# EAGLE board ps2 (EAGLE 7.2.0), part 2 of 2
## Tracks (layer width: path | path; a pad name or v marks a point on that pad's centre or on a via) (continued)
KNOCKER+ (continued)
  Top 0.254: R18.1 99.21,12.23 100.36,12.23 103.33,15.2 114.19,15.2 115.67,13.72 R45.2
  Bottom 0.254: OK7.1 121.16,22.06 117.16,18.06 117.16,15.09 115.79,13.72 R45.2
KNOCKER-  (via drill 0.61)
  Top 0.254: 124.3,14.92 123.1,13.72 R48.1 | 124.3,14.92 127.33,17.95 127.33,24.12 126.64,24.8 125.84,24.8 125.62,24.57 120.81,24.57 119.79,25.6 118.64,25.6 OK7.2 | v8.12,27.77 6.63,29.26 6.63,34.4 2.63,38.41 2.63,38.86 T3.C | v31.77,15.66 33.15,15.09 50.41,15.09 54.41,11.09 66.75,11.09 67.32,11.66 67.32,14.4 65.95,15.77 64.35,15.77 63.78,16.46 63.78,18.75 64.81,19.77 69.84,19.77 73.15,16.46 73.15,12 76.35,8.8 76.35,5.83 v77.84,4.34 | v96.24,4.34 99.44,4.34 99.61,4.17 | 99.61,4.17 101.73,2.06 R10.2 | v99.67,4.23 99.61,4.17 | 124.3,14.92 127.67,11.54 v127.67,11.43 | v121.84,8.91 121.84,11.09 120.93,12 113.96,12 112.47,10.52 C9.2
  Bottom 0.254: v8.12,27.77 11.2,24.69 22.75,24.69 v31.77,15.66 | v96.24,4.34 v77.84,4.34 | v99.67,4.23 102.3,6.86 112.81,6.86 113.39,7.43 113.39,8.34 112.47,9.26 112.47,10.4 C9.2 | v127.67,11.43 127.1,11.43 124.24,8.57 122.19,8.57 v121.84,8.91
KNOCKER_TRIGGER  (via drill 0.61)
  Top 0.254: v18.63,68.01 18.63,77.15 20.8,79.32 21.83,79.32 22.75,78.41 22.75,77.72 23.66,76.81 24.35,76.81 v26.86,74.3 | v30.29,64.58 31.77,63.09 31.77,59.44 33.26,57.95 FRDM1.D6
  Bottom 0.254: v18.63,68.01 15.66,65.04 15.66,54.86 12.46,51.66 12.46,47.43 R37.1 | v26.86,74.3 26.86,70.98 30.29,67.55 v30.29,64.58
MOSFETIN2
  Top 0.254: IC2.4 100.36,23.66 111.56,23.66 113.5,25.6 OK7.4
MOSFETIN3
  Top 0.254: OK7.6 108.36,25.6 107.33,25.6 106.3,24.57 101.84,24.57 100.36,26.06 IC2.5
MOSFETIN4
  Top 0.254: IC2.6 100.36,28.69 103.33,25.72 OK7.8
MOSFETIN5
  Top 0.254: IC2.7 100.36,31.32 105.16,31.32 107.21,33.38 114.41,33.38 118.53,37.49 OK8.2
MOSFETIN6
  Top 0.254: OK8.4 109.84,33.83 100.36,33.83 IC2.8
MOSFETIN7
  Top 0.254: IC2.9 100.36,36.35 107.21,36.35 108.36,37.49 OK8.6
MOSFETIN8
  Top 0.254: IC2.10 102.07,38.86 103.33,37.6 OK8.8
MOSFETIN9
  Top 0.254: IC2.11 100.36,41.49 101.61,41.49 103.67,43.55 107.44,43.55 112.24,48.35 117.5,48.35 118.53,49.38 OK9.2
MOSFETIN10
  Top 0.254: IC2.12 100.36,44.01 107.21,44.01 112.58,49.38 113.5,49.38 OK9.4
MOSFETIN11
  Top 0.254: IC2.13 100.36,46.52 105.5,46.52 108.36,49.38 OK9.6
MOSFETIN12
  Top 0.254: IC2.14 100.36,49.03 102.98,49.03 103.33,49.38 OK9.8
MOSFETIN13  (via drill 0.61)
  Top 0.254: v101.04,52.46 100.24,51.66 95.56,51.66 IC2.15
  Bottom 0.254: v101.04,52.46 102.3,53.72 102.3,58.86 104.93,61.49 104.93,66.06 105.5,66.64 116.59,66.64 117.61,65.61 117.61,62.41 118.53,61.49 OK10.2
MOSFETIN14  (via drill 0.61)
  Top 0.254: v106.07,59.66 101.73,55.32 99.67,55.32 96.47,52.12 94.18,52.12 92.81,53.49 92.81,53.84 IC3.28
  Bottom 0.254: v106.07,59.66 111.78,59.66 113.5,61.38 OK10.4
MOSFETIN15
  Top 0.254: IC3.1 100.36,53.95 101.61,53.95 108.36,60.69 108.36,61.38 OK10.6
MOSFETIN16
  Top 0.254: IC3.2 100.36,56.46 100.36,56.81 103.33,59.78 103.33,61.38 OK10.8
MOSFETIN17
  Bottom 0.254: IC3.3 100.36,58.98 100.36,59.32 102.3,61.27 102.3,66.06 104.93,68.69 113.96,68.69 118.53,73.27 OK11.2
MOSFETIN18  (via drill 0.61)
  Top 0.254: v102.64,68.01 102.64,68.58 104.93,70.87 104.93,77.95 105.96,78.98 110.98,78.98 112.47,77.5 112.47,74.3 113.5,73.27 OK11.4
  Bottom 0.254: v102.64,68.01 99.67,68.01 98.64,66.98 98.64,63.55 100.24,61.95 100.24,61.49 IC3.4
MOSFETIN19
  Top 0.254: IC3.5 100.36,64.01 100.36,64.47 107.67,71.78 107.67,72.58 108.36,73.27 OK11.6
MOSFETIN20
  Top 0.254: IC3.6 100.36,66.64 100.36,66.98 103.33,69.95 103.33,73.27 OK11.8
MOSFETIN21
  Bottom 0.254: IC3.7 100.36,69.15 108.36,69.15 112.47,73.27 112.47,78.3 118.53,84.35 118.53,85.04 OK12.2
MOSFETIN22
  Bottom 0.254: IC3.8 100.36,71.67 103.21,71.67 104.47,72.92 104.47,79.9 107.56,82.98 111.44,82.98 113.5,85.04 OK12.4
MOSFETIN23
  Top 0.254: IC3.9 100.36,74.18 100.36,74.64 102.3,76.58 102.3,78.41 108.36,84.47 108.36,85.04 OK12.6
MOSFETIN24
  Top 0.254: IC3.10 100.36,76.81 100.36,77.15 105.73,82.53 105.73,83.67 104.24,83.67 OK12.8
MOSFETOUT1  (via drill 0.61)
  Top 1.575: Q7A.2 145.03,6.86 150.53,12.8 v150.53,15.54
  Bottom 1.575: v150.53,15.54 153.28,18.75 JP10.1
MOSFETOUT2
  Bottom 1.575: Q7B.2 130.81,5.71 130.81,9.53 136.53,9.53 137.16,10.16 137.16,13.34 136.53,13.97 136.53,16.51 148.59,16.51 150.42,18.52 JP10.2
MOSFETOUT3
  Bottom 1.575: Q7C.2 144.15,9.53 147.71,9.53 149.39,11.54 152.82,15.2 153.62,16.12 155.87,18.82 155.87,20.79 154.42,22.05 JP10.3
MOSFETOUT4
  Bottom 1.575: Q7D.2 130.81,13.97 130.81,18.41 147.32,18.41 150.72,22.16 151.36,22.16 JP10.4
MOSFETOUT5
  Top 1.575: Q8A.2 141.6,20.95 141.6,19.68 143.51,17.78 154.94,17.78 156.21,19.05 156.21,22.86 154.31,24.77 JP10.5
MOSFETOUT6
  Bottom 1.575: Q8B.2 128.91,22.86 128.91,25.4 150.5,25.4 151.13,24.77 JP10.6
MOSFETOUT7  (via drill 0.61)
  Top 1.575: v156.21,35.56 156.21,29.21 154.31,27.3 JP10.7 | v144.15,36.83 140.97,33.66 140.97,30.48 Q8C.2
  Bottom 1.575: v156.21,35.56 154.94,36.83 v144.15,36.83
MOSFETOUT8
  Bottom 1.575: Q8D.2 128.91,31.75 128.91,27.3 151.13,27.3 JP10.8
MOSFETOUT9
  Bottom 1.575: Q9A.2 141.48,34.92 154.31,34.92 156.21,33.02 156.21,29.84 154.31,29.84 JP10.9
MOSFETOUT10  (via drill 0.61)
  Top 1.575: v142.88,33.02 144.78,34.92 147.32,34.92 148.34,33.66 148.34,31.75 149.99,29.84 151.13,29.84 JP10.10
  Bottom 1.575: v142.88,33.02 139.06,33.02 134.62,37.47 132.72,37.47 128.78,40.77 Q9B.2
MOSFETOUT11
  Top 1.575: JP10.11 153.9,32.61 153.96,33.83 151.02,37.21 150.77,37.71 150.75,47.12 149.61,49.02 146.94,49.02 146.05,47.37 143.89,46.35 141.48,47.75 Q9C.2
MOSFETOUT12  (via drill 0.61)
  Top 1.575: v148.48,41.47 148.48,36.8 151.33,33.38 151.36,32.5 JP10.12
  Bottom 1.575: v148.48,41.47 148.46,43.56 147.83,44.83 146.3,44.83 144.91,46.61 132.21,46.61 128.78,49.91 Q9D.2
MOSFETOUT13
  Top 1.575: Q10A.2 156.21,46.99 155.57,46.99 152.4,50.16 152.4,57.15 154.31,59.05 JP11.1
MOSFETOUT14
  Top 1.575: Q10B.2 141.6,57.78 141.6,57.15 143.51,55.24 147.32,55.24 151.13,59.05 JP11.2
MOSFETOUT15  (via drill 0.61)
  Top 1.575: v154.31,55.24 156.21,57.15 156.21,60.33 154.31,62.23 JP11.3
  Bottom 1.575: v154.31,55.24 128.91,55.24 128.91,59.69 Q10C.2
MOSFETOUT16
  Bottom 1.575: JP11.4 151.13,62.23 147.32,62.23 146.69,62.87 133.99,62.87 128.91,67.94 128.91,69.22 Q10D.2
MOSFETOUT17  (via drill 0.61)
  Top 1.575: v147.96,59.69 147.96,61.59 144.78,64.77 v138.89,64.77
  Bottom 1.575: v147.96,59.69 150.5,57.15 156.21,57.15 156.21,62.23 154.31,64.14 JP11.5 | Q11A.2 128.84,76.33 132.72,73.03 133.35,72.45 133.35,69.85 133.39,69.85 133.39,69.72 135.56,67.44 135.56,65.95 136.82,64.81 v138.89,64.77
MOSFETOUT18
  Bottom 1.575: JP11.6 151.13,64.77 143.51,64.77 141.48,66.29 Q11B.2
MOSFETOUT19  (via drill 0.61)
  Top 1.575: v149.22,75.56 147.32,75.56 144.78,73.03 143.51,73.03 141.48,75.18 Q11C.2
  Bottom 1.575: v149.22,75.56 149.86,74.93 156.21,74.93 156.21,68.58 154.94,67.31 154.31,67.31 JP11.7
MOSFETOUT20
  Bottom 1.575: Q11D.2 128.79,84.99 128.79,83.96 132.08,80.64 133.99,78.74 133.99,76.83 134.62,76.83 139.7,71.75 147.32,71.75 149.22,69.85 149.22,67.31 151.13,67.31 JP11.8
MOSFETOUT21  (via drill 0.61)
  Top 1.575: Q12A.2 144.78,92.08 v149.22,87.63 | v154.94,76.83 156.21,75.56 156.21,71.12 154.31,69.22 JP11.9
  Bottom 1.575: v149.22,87.63 149.22,80.64 150.5,79.38 150.5,76.83 v154.94,76.83
MOSFETOUT22  (via drill 0.61)
  Top 1.575: v146.69,92.71 151.13,88.27 151.13,74.3 149.22,72.39 149.22,71.12 151.13,69.22 JP11.10
  Bottom 1.575: Q12B.2 131.44,92.71 v146.69,92.71
MOSFETOUT23  (via drill 0.61)
  Top 1.575: v153.03,78.74 153.03,76.2 153.67,75.56 153.67,72.39 JP11.11
  Bottom 1.575: v153.03,78.74 152.4,79.38 152.4,85.09 Q12C.2
MOSFETOUT24
  Bottom 1.575: Q12D.2 141.6,85.09 141.6,80.64 146.69,80.64 147.96,79.38 147.96,76.83 147.32,76.2 147.32,73.66 148.59,73.66 149.86,72.39 151.13,72.39 JP11.12
N$1  (via drill 0.61)
  Top 0.254: v96.24,24.57 96.24,33.03 93.95,35.32 89.72,35.32 89.15,35.89 89.15,36.69 88.47,37.38 86.75,37.38 80.24,43.89 79.78,43.89 IC1.17
  Bottom 0.254: v96.24,24.57 92.81,21.14 IC2.26
N$2
  Top 0.254: IC2.17 92.7,44.01 91.21,44.01 89.15,46.06 89.15,50.98 90.53,52.35 90.53,56.69 92.7,58.86 IC3.26
N$3  (via drill 0.61)
  Top 0.254: v83.67,56.01 83.67,67.44 83.78,67.55 83.78,74.3 v83.33,74.75 | v95.33,79.32 95.33,80.58 94.18,81.72 92.81,81.72 IC3.17
  Bottom 0.254: v83.67,56.01 80.81,58.86 79.78,58.86 IC4.26 | v83.33,74.75 86.3,77.72 93.73,77.72 v95.33,79.32
N$4
  Bottom 0.254: R18.2 99.21,2.06 99.21,2.52 103.1,6.4 114.07,6.4 117.96,10.29 IC11.3
N$5
  Top 0.254: OK15.1 16.92,70.29 15.89,70.29 14.86,69.27 14.06,69.27 12,71.32 12,71.55 R39.1
N$6  (via drill 0.61)
  Top 0.254: v103.44,4.23 102.41,5.26 95.9,5.26 95.33,4.69 95.33,4 96.58,2.74 96.58,2.06 R6.1 | IC11.4 115.44,10.29 113.73,10.29 112.36,8.91 112.01,8.91 106.98,3.89 C5.+
  Bottom 0.254: v103.44,4.23 106.64,4.23 C5.+
N$8  (via drill 0.61)
  Top 0.254: v2.86,70.75 2.86,68.69 1.26,67.09 1.26,32.92 4.34,29.83 4.34,25.95 2.06,23.66 R38.1 | v2.86,83.33 2.86,85.84 1.83,86.87 R47.2 1.83,86.98 1.83,87.55 10.74,96.47 10.74,96.93 T5.C
  Bottom 0.254: v2.86,83.33 v2.86,70.75
N$9
  Bottom 0.254: R37.2 2.63,45.83 5.03,43.55 5.03,38.86 T3.B
N$10
  Top 0.254: OK13.1 10.97,26.4 10.97,24.8 12.12,23.66 R38.2
N$11
  Top 0.254: R49.2 12,69.04 12,65.15 14.4,62.75 OK15.3
N$12
  Bottom 0.254: T6.B 5.03,33.72 4.57,33.72 2.97,32.12 2.06,32.12 1.26,32.92 1.26,68.58 1.71,69.04 R49.1
N$13
  Top 0.254: R44.2 1.83,79.32 1.83,79.78 8.8,86.75 8.8,92.47 10.74,94.41 T5.B
N$14
  Top 0.254: R44.1 12,79.32 12,81.72 R41.1 12,81.84 12,82.87 17.49,88.35 17.49,94.53 15.43,96.58 15.43,96.93 T4.C
N$15  (via drill 0.61)
  Top 0.254: v30.52,20.34 31.77,20.34 32.58,19.55 32.58,16.92 33.72,15.54 50.63,15.54 54.18,12 v66.41,12 | v83.21,12.34 91.78,12.34 D1.A
  Bottom 0.254: v30.52,20.34 22.29,28.57 16.92,28.57 10.06,35.43 4.57,35.43 2.97,33.83 2.63,33.83 T6.C | v66.41,12 71.32,12 73.5,9.83 K1.16 73.61,9.83 74.87,11.09 81.95,11.09 v83.21,12.34
N$16
  Top 0.254: K1.4 81.15,2.29 76.81,6.63 76.81,13.03 JP9.2
N$17
  Top 0.254: R2.1 77.04,36.35 79.67,36.35 IC1.20
N$18
  Top 0.254: R3.1 90.18,36.35 92.7,36.35 IC2.20
N$19
  Top 0.254: R4.1 89.95,74.18 92.7,74.18 IC3.20
N$20
  Top 0.254: R5.1 77.27,74.18 79.67,74.18 IC4.20
N$21
  Bottom 0.254: FRDM1.A0 35.78,9.6 35.78,6.06 35.55,5.83 35.55,2.4 36.35,1.6 56.81,1.6 59.44,4.23 66.06,4.23 67.21,5.37 JP7.1
N$22  (via drill 0.61)
  Top 0.254: v55.78,21.14 49.15,21.14 44.46,25.83 44.01,25.83 IC5.3
  Bottom 0.254: v55.78,21.14 58.64,18.29 58.64,16.57 59.78,15.43 64.69,15.43 67.21,17.95 67.21,18.29 OK1.15
N$23
  Bottom 0.254: OK1.13 61.15,18.29 55.44,24 38.18,24 36.35,25.83 IC5.6
N$24
  Top 0.254: IC5.11 36.69,18.29 38.41,16.57 41.83,16.57 42.86,17.6 42.86,19.32 44.01,20.46 51.32,20.46 53.61,18.17 53.61,16.46 54.18,15.89 54.98,15.89 57.15,18.06 OK1.11
N$25
  Top 0.254: IC5.14 44.35,18.29 46.06,20 50.29,20 52.01,18.29 OK1.9
N$26
  Top 0.254: FRDM1.PTE20 35.89,12.23 36.46,12.23 38.86,14.63 50.06,14.63 56.81,7.89 64.01,7.89 65.95,5.94 65.95,2.17 65.27,1.6 64.12,1.6 63.44,2.29 63.44,3.43 62.64,4.23 61.27,4.23 JP7.8
N$27  (via drill 0.61)
  Top 0.254: v57.49,34.75 47.43,34.75 44.35,37.83 44.01,37.83 IC6.3 | v66.06,32.69 66.06,32.12 67.21,30.98 67.21,30.29 OK2.15
  Bottom 0.254: v57.49,34.75 58.06,34.75 60.12,32.69 v66.06,32.69
N$28  (via drill 0.61)
  Top 0.254: v56.58,33.83 v48.12,33.83
  Bottom 0.254: v48.12,33.83 40.8,33.83 36.8,37.83 36.35,37.83 IC6.6 | v56.58,33.83 58.29,33.83 61.84,30.29 62.18,30.29 OK2.13
N$29  (via drill 0.61)
  Top 0.254: v45.26,32.35 55.09,32.35 57.15,30.29 OK2.11
  Bottom 0.254: v45.26,32.35 38.86,32.35 36.8,30.29 36.35,30.29 IC6.11
N$30
  Top 0.254: OK2.9 50.41,31.89 46.06,31.89 44.46,30.29 44.01,30.29 IC6.14
N$31  (via drill 0.61)
  Top 0.254: v48.35,44.12 48.35,45.38 IC7.3
  Bottom 0.254: v48.35,44.12 54.06,44.12 55.66,42.52 55.66,37.83 59.44,34.06 65.38,34.06 65.95,34.63 65.95,39.32 67.21,40.58 67.21,42.06 OK3.15
N$32
  Bottom 0.254: OK3.13 62.18,42.18 61.15,42.18 57.38,45.95 40.12,45.95 36.35,49.72 IC7.6
N$33  (via drill 0.61)
  Top 0.254: v37.26,45.95 36.35,45.03 36.35,42.18 IC7.11
  Bottom 0.254: v37.26,45.95 39.43,45.95 39.89,45.49 56.69,45.49 57.26,44.92 57.26,42.29 57.15,42.18 OK3.11
N$34
  Top 0.254: FRDM1.PTE21 38.41,12.23 38.98,12.23 40.92,14.17 49.84,14.17 56.58,7.43 62.75,7.43 64.69,5.49 JP7.3
N$35
  Bottom 0.254: IC7.14 44.01,42.06 44.46,42.06 46.06,40.46 50.41,40.46 52.01,42.06 OK3.9
N$36
  Top 0.254: IC8.3 42.98,70.18 43.43,70.18 45.03,71.78 50.06,71.78 57.84,64.01 68.01,64.01 69.49,62.52 OK4.15
N$37
  Bottom 0.254: OK4.13 64.35,62.52 63.32,62.52 57.72,68.12 53.49,68.12 52.46,67.09 38.29,67.09 35.32,70.07 IC8.6
N$38
  Top 0.254: JP6.2 50.86,4 50.86,5.6 49.95,6.51 49.72,6.51 47.43,8.8 47.43,10.17 46.06,11.54 46.06,12.12 FRDM1.PTE29
N$39  (via drill 0.61)
  Top 0.254: v48.58,59.89 37.6,59.89 35.32,62.18 35.32,62.41 IC8.11
  Bottom 0.254: v48.58,59.89 57.04,59.89 59.32,62.18 59.32,62.41 OK4.11
N$40
  Bottom 0.254: OK4.9 52.58,60.81 45.03,60.81 43.43,62.41 42.98,62.41 IC8.14
N$41
  Bottom 0.254: R42.1 12.46,42.18 12.8,42.18 13.6,43.43 16,43.43 17.83,41.26 17.83,38.86 27.66,30.18 27.66,26.06 28.57,25.26 28.92,25.26 33.38,20.92 36.01,20.92 37.38,19.55 37.38,17.03 40.69,13.95 41.15,13.95 42.75,12.23 43.43,12.23 FRDM1.PTE23
N$42
  Top 0.254: 128.13,5.49 124.36,9.26 124.36,11.2 123.56,12 122.53,12 122.07,12.46 118.07,12.46 117.27,13.26 117.27,13.72 113.61,17.37 113.61,17.95 OK7.13 | 128.13,5.49 125.62,2.97 R7.2 | 128.13,5.49 Q7B.1
N$43
  Bottom 0.254: 2.86,84.24 1.83,84.24 R40.1 | 2.86,84.24 3.2,84.24 9.26,78.18 11.89,78.18 14.4,75.67 14.4,74.98 OK14.3 | 2.86,84.24 2.86,87.21 1.83,88.24 1.83,89.38 R46.2
N$44
  Top 0.254: 144.02,30.52 Q8C.1
  Bottom 0.254: OK8.11 108.47,29.95 109.61,29.95 113.84,34.18 132.93,34.18 138.53,28.57 142.19,28.57 144.02,30.4 Q8C.1 144.13,30.52 146.3,32.69 R9.2
N$45
  Top 0.254: OK8.9 103.44,29.95 104.47,29.95 105.96,31.43 121.96,31.43 123.56,29.83 R22.2 123.67,29.72 126.19,32.23 Q8D.1 126.3,32.23
N$46
  Top 0.254: R19.2 146.42,23.43 144.02,21.03 Q8A.1 144.02,20.92
  Bottom 0.254: OK8.15 118.64,29.95 119.79,29.95 120.81,30.98 121.5,30.98 122.53,29.95 122.53,28.92 127.56,23.89 127.56,21.72 128.36,20.92 132.7,20.92 134.19,22.4 138.07,22.4 138.53,22.86 142.19,22.86 144.02,21.03 Q8A.1
N$47
  Top 0.254: OK8.13 113.61,29.83 113.61,28.35 114.99,26.98 114.99,25.26 119.9,20.34 123.33,20.34 R20.2 123.44,20.34 123.67,20.34 126.19,22.86 Q8B.1 126.3,22.86
N$48
  Top 0.254: Q7D.1
  Bottom 0.254: Q7D.1 125.62,11.2 125.39,11.2 R24.2 125.27,11.2 124.47,12 115.33,12 112.13,15.2 105.96,15.2 103.44,17.72 103.44,17.95 OK7.9
N$49
  Top 0.254: R26.2 148.7,14.63 148.7,14.17 146.76,12.23 Q7C.1 146.65,12.23
  Bottom 0.254: Q7C.1 144.82,14.06 141.16,14.06 140.47,13.37 140.47,11.89 136.93,8.34 133.73,8.34 132.13,6.74 132.13,4.57 131.1,3.54 130.19,3.54 129.5,4.23 129.5,14.74 128.59,15.66 127.67,15.66 124.7,12.69 115.33,12.69 112.36,15.66 110.64,15.66 109.96,16.34 109.96,16.46 108.47,17.95 OK7.11
N$50
  Top 0.254: JP9.1 76.81,15.54 76.81,14.63 78.18,13.26 78.18,10.97 85.72,3.43 89.95,3.43 91.21,2.17 K1.8
N$51
  Top 0.254: 144.02,40.35 Q9A.1
  Bottom 0.254: OK9.15 118.64,41.83 119.79,41.83 122.07,44.12 140.36,44.12 144.02,40.46 Q9A.1 144.13,40.46 146.53,42.86 R11.2
N$52
  Top 0.254: 124.3,40.18 126.19,42.06 Q9B.1 126.3,42.18 | 124.3,40.18 123.79,39.66 123.44,39.66 R13.2 | 124.3,40.18 121.16,43.32 116.13,43.32 114.64,41.83 113.61,41.83 OK9.13
N$53  (via drill 0.61)
  Top 0.254: v127.44,53.38 127.44,49.95 124.93,47.43 117.73,47.43 112.47,42.18 112.47,37.49 111.44,36.46 110.64,36.46 109.96,37.15 109.96,38.86 108.47,40.35 108.47,41.72 OK9.11 | 144.02,49.26 Q9C.1
  Bottom 0.254: v127.44,53.38 138.76,53.38 140.93,51.21 142.19,51.21 144.02,49.38 Q9C.1 144.13,49.38 146.53,51.78 R15.2
N$54
  Top 0.254: 126.3,51.09 Q9D.1 126.19,50.98 125.96,50.98 123.56,48.58 R17.2 123.44,48.46 122.87,47.89 112.47,47.89 107.67,43.09 105.73,43.09 104.47,41.83 103.44,41.83 OK9.9
N$55  (via drill 0.61)
  Top 0.254: R21.2 154.08,51.55 154.42,51.55 156.59,49.38 Q10A.1 | v139.33,51.55 145.39,51.55 146.76,50.18 150.76,50.18 155.45,45.49 157.73,45.49 158.53,46.29 158.53,47.43 156.71,49.26 Q10A.1 | 156.59,49.26 Q10A.1
  Bottom 0.254: v139.33,51.55 137.96,52.92 128.25,52.92 127.56,52.23 127.56,50.06 126.64,49.15 125.73,49.15 125.04,49.84 125.04,51.32 121.5,54.86 120.81,54.86 119.79,53.84 118.64,53.84 OK10.15
N$56  (via drill 0.61)
  Top 0.254: v139.68,53.72 139.68,56.69 140.25,57.26 140.25,59.44 141.05,60.24 142.07,60.24 Q10B.1
  Bottom 0.254: v139.68,53.72 139.56,53.84 128.7,53.84 127.22,55.32 116.13,55.32 114.64,53.84 113.61,53.84 OK10.13 | R23.2 146.3,60.58 Q10B.1
N$57
  Top 0.254: 126.3,59.89 Q10C.1 123.67,57.38 123.56,57.38 R25.2 123.44,57.38 113.16,57.38 109.61,53.84 108.47,53.84 OK10.11
N$58
  Top 0.254: 126.3,69.38 Q10D.1 126.19,69.27 125.96,69.27 123.56,66.86 R27.2 123.44,61.49 121.16,59.21 109.84,59.21 104.47,53.84 103.44,53.84 OK10.9
N$59
  Top 0.254: 126.3,77.72 Q11A.1 126.19,77.61 125.62,77.61 R28.2 123.1,75.09 123.1,73.72 118.64,69.27 118.64,65.72 OK11.15
N$60  (via drill 0.61)
  Top 0.254: v144.82,60.35 145.28,60.35 147.1,58.52 148.48,58.52 149.16,59.21 149.16,62.41 Q11B.1 144.02,67.78 146.3,70.07 R29.2
  Bottom 0.254: v144.82,60.35 138.65,60.35 138.07,59.78 135.56,59.78 133.5,61.84 125.73,61.84 124.24,60.35 115.67,60.35 114.99,61.04 114.99,62.75 113.61,64.12 113.61,65.61 OK11.13
N$61
  Top 0.254: R36.2 12,76.81 12,77.84 14.4,80.24 14.4,82.53 OK14.2
N$62  (via drill 0.61)
  Top 0.254: v124.7,69.27 124.47,69.27 122.42,67.21 122.42,61.15 120.93,59.66 111.21,59.66 109.96,60.92 109.96,62.64 108.47,64.12 108.47,65.61 OK11.11 | 144.02,76.12 Q11C.1
  Bottom 0.254: v124.7,69.27 124.7,82.98 127.56,85.84 127.56,88.01 128.36,88.81 129.16,88.81 130.19,87.78 130.19,84.58 135.1,79.67 140.47,79.67 144.02,76.12 Q11C.1 144.02,76.24 146.3,78.52 R30.2
N$63  (via drill 0.61)
  Top 0.254: v108.58,71.89 103.44,66.75 103.44,65.72 OK11.9 | v115.44,83.44 122.3,83.44 R31.2
  Bottom 0.254: v108.58,71.89 109.96,73.27 109.96,77.95 v115.44,83.44 | R31.2 125.62,86.87 Q11D.1
N$64
  Top 0.254: R32.2 149.05,97.84 149.05,97.16 147.33,95.44 Q12A.1 147.33,95.33
  Bottom 0.254: OK12.15 118.53,77.5 118.53,76.01 117.16,74.64 117.16,72.92 116.47,72.24 115.67,72.24 114.99,72.92 114.99,77.84 121.27,84.12 121.61,84.12 122.19,84.7 122.19,85.15 128.59,91.55 147.22,91.55 147.9,92.24 147.9,94.75 147.33,95.33 Q12A.1
N$65
  Top 0.254: 128.93,97.16 Q12B.1
  Bottom 0.254: OK12.13 113.61,77.61 113.61,78.64 120.13,85.15 120.13,88.7 126.42,94.98 R33.2 126.53,94.98 126.64,94.98 128.82,97.16 Q12B.1
N$66  (via drill 0.61)
  Top 0.254: 157.05,87.67 Q12C.1 R34.2 | v109.04,67.78 109.5,68.24 109.5,74.98 108.47,76.01 108.47,77.5 OK12.11 | v119.56,66.98 119.56,68.69 127.67,76.81 127.67,83.33 v131.44,84.58
  Bottom 0.254: v109.04,67.78 118.76,67.78 v119.56,66.98 | v131.44,84.58 137.5,90.64 153.96,90.64 R34.2
N$67  (via drill 0.61)
  Top 0.254: 144.02,85.04 Q12D.1 144.13,85.15 144.13,85.38 146.3,87.55 R35.2 146.3,87.67 143.56,90.41 143.56,96.47 142.76,97.27 v141.28,97.27 | v122.64,94.53 124.36,94.53 125.96,96.13 127.56,96.13 128.47,95.21 v133.04,95.21
  Bottom 0.254: v122.64,94.53 121.39,93.27 118.87,93.27 112.47,86.87 112.47,85.15 110.76,83.44 107.33,83.44 103.44,79.55 103.44,77.61 OK12.9 | v133.04,95.21 135.1,95.21 136.82,96.93 140.93,96.93 v141.28,97.27
N$68  (via drill 0.61)
  Top 0.254: C1.2 77.72,33.83 79.67,33.83 IC1.21 | IC1.27 79.67,18.63 77.04,18.63 R1.2 77.04,18.75 77.04,19.43 72.92,23.55 72.92,29.95 C6.2 72.81,30.06 72.81,33.83 72.69,33.95 C10.- | C4.2 77.72,71.67 79.67,71.67 IC4.21 | IC4.19 79.78,76.69 79.78,76.24 81.5,74.52 81.5,73.61 79.67,71.78 IC4.21 | IC2.27 92.81,18.63 92.81,19.09 94.87,21.14 94.87,31.66 92.81,33.72 IC2.21 92.7,33.83 90.75,33.83 C2.2 | 83.5,48.06 85.04,46.52 85.04,44.12 86.75,42.41 88.47,42.41 89.72,41.15 89.72,38.98 90.3,38.41 92.24,38.41 92.7,38.86 IC2.19 | 83.5,48.06 81.61,49.95 81.61,54.06 79.78,55.89 79.78,56.35 IC4.27 | 91.67,60.01 93.73,60.01 94.41,59.32 94.41,58.52 92.81,56.92 92.81,56.46 IC3.27 | 91.67,60.01 89.5,57.84 89.5,53.84 87.21,51.55 86.98,51.55 83.5,48.06 | v90.64,66.29 90.64,61.15 91.67,60.12 91.67,60.01 | v82.41,68.12 82.41,68.58 79.78,71.21 79.78,71.55 IC4.21
  Bottom 0.254: 77.95,35.2 77.95,34.06 77.72,33.83 C1.2 | 77.95,35.2 77.95,36.69 79.67,38.41 79.67,38.86 IC1.19 | 77.95,35.2 73.84,35.2 72.69,34.06 C10.- | IC12.2 73.15,87.55 71.21,85.61 71.21,82.98 C11.+ 73.27,81.04 77.5,76.81 79.67,76.81 IC4.19 | C3.2 89.95,71.67 92.7,71.67 IC3.21 | IC3.19 92.81,76.69 92.81,76.24 94.41,74.64 94.41,73.5 92.7,71.78 IC3.21 | IC3.21 92.81,71.55 92.81,71.09 94.41,69.49 94.41,68.69 93.27,67.55 91.55,67.55 90.64,66.64 v90.64,66.29 90.53,66.64 89.61,67.55 86.75,67.55 86.18,68.12 v82.41,68.12 | IC2.21 92.81,33.83 92.81,34.29 94.41,35.89 94.41,37.26 92.81,38.86 IC2.19 | IC1.21 79.78,33.83 81.04,35.2 89.27,35.2 90.64,33.83 C2.2
N$69
  Top 0.254: C7.1 112.47,2.63 115.44,2.63 IC11.5
N$70  (1 unrouted)
  Top 0.254: JP4.3 JP4.2
N$71
  Top 0.254: IC11.7 120.47,2.74 118.07,2.74 IC11.6 117.96,2.74 117.5,2.74 115.79,4.46 113.27,4.46 112.36,3.54 110.98,3.54 109.39,1.94 104.36,1.94 R8.2 104.36,2.06 104.36,6.51 106.98,9.14 C8.+ 106.98,9.26 106.64,9.6 106.64,13.37 T2.E
N$72  (via drill 0.61)
  Top 0.254: v134.53,7.43 130.42,7.43 126.76,11.09 126.76,11.2 125.5,12.46 122.76,12.46 121.96,13.26 121.96,13.72 118.64,17.03 118.64,17.95 OK7.15 | 147.56,2.63 Q7A.1
  Bottom 0.254: v134.53,7.43 142.88,7.43 147.1,3.2 | 147.1,3.2 147.56,2.74 Q7A.1 147.1,3.2 | 147.1,3.2 149.05,5.14 R14.2
N$73
  Top 0.254: IC9.3 43.32,82.3 48.81,76.81 64.24,76.81 66.29,74.75 OK5.15
N$74
  Top 0.254: IC11.2 120.47,10.29 120.02,10.29 117.61,7.89 112.47,7.89 C9.1
  Bottom 0.254: 108.47,7.77 112.36,7.77 C9.1 | 108.47,7.77 100.93,7.77 95.21,2.06 94.18,2.06 R12.2 | 108.47,7.77 108.47,9.72 109.04,10.29 109.04,13.37 T2.B
N$75
  Top 0.254: JP7.4 64.69,3.66 63.55,4.69 63.55,5.6 62.18,6.97 56.35,6.97 49.61,13.72 42.98,13.72 41.49,12.23 40.92,12.23 FRDM1.PTE22
N$76
  Top 0.254: IC4.17 79.67,81.72 79.67,81.27 75.67,77.27 75.67,64.47 76.12,64.01 JP12.6
N$77
  Bottom 0.254: OK5.13 61.15,74.75 60.01,74.75 54.18,80.58 37.03,80.58 IC9.6
N$78
  Bottom 0.254: IC9.11 35.32,74.75 35.78,74.75 37.38,76.35 43.32,76.35 44.46,75.21 44.46,73.61 45.15,72.92 48.35,72.92 50.06,74.64 50.06,77.95 50.75,78.64 52.23,78.64 56.12,74.75 OK5.11
N$79
  Top 0.254: OK5.9 49.38,76.35 45.03,76.35 43.43,74.75 42.98,74.75 IC9.14
N$80
  Top 0.254: IC10.3 48.81,88.35 63.44,88.35 65.15,86.64 66.29,86.64 OK6.15
N$81  (via drill 0.61)
  Top 0.254: v37.95,89.95 35.32,92.58 35.32,94.18 IC10.6
  Bottom 0.254: v37.95,89.95 38.86,90.3 57.49,90.3 61.15,86.64 OK6.13
N$82
  Bottom 0.254: IC10.11 35.32,86.64 35.78,86.64 37.49,88.35 54.41,88.35 56.12,86.64 OK6.11
N$83
  Top 0.254: IC10.14 42.98,86.53 43.43,86.53 45.03,84.92 49.38,84.92 50.98,86.53 OK6.9
N$85
  Top 0.254: R40.2 12,84.35 12,86.87 R47.1 12.46,86.87 17.03,91.44 17.03,92.35 15.43,93.95 15.43,94.41 T4.B
N$86  (via drill 0.61)
  Top 0.254: v79.55,13.26 79.55,12.8 81.27,11.09 89.95,11.09 91.21,9.83 K1.9
  Bottom 0.254: v79.55,13.26 78.98,13.26 77.72,12 76.24,12 75.21,13.03 74.3,13.03 JP9.4
N$87
  Top 0.254: JP9.3 74.3,15.66 75.21,15.66 76.35,16.8 77.27,16.8 78.07,16 78.07,14.06 78.64,13.49 78.64,12.34 81.15,9.83 K1.13
N$88
  Bottom 0.457: JP6.3 R43.2
N$89  (via drill 0.61)
  Top 0.254: v35.2,16.46 35.78,16 51.09,16 52.12,14.97 v54.63,14.97
  Bottom 0.254: JP6.1 57.15,12.34 57.15,14.06 56.35,14.97 v54.63,14.97 | T1.C 9.72,37.6 14.4,32.92 20.46,32.92 26.75,26.86 26.75,26.18 30.75,21.95 31.2,21.95 33.15,20.12 34.52,20.12 35.2,19.43 v35.2,16.46
N$100
  Top 0.254: R42.2 2.29,42.63 9.14,42.63 12.23,39.32 T1.B
PSU2_STATUS_SENSE  (via drill 0.61)
  Top 0.254: R16.2 1.83,74.07 1.83,73.72 13.49,62.06 13.49,60.92 14.97,59.44 17.72,59.44 19.2,57.95 FRDM1.D11 19.2,57.84 18.17,56.81 18.17,54.86 17.72,54.41 v17.72,27.66
  Bottom 0.254: v17.72,27.66 10.74,27.66 9.49,28.92 3.31,28.92 OK13.3
PSU2_STATUS_SET
  Bottom 0.254: OK14.1 16.92,82.53 16.92,78.64 15.54,77.27 15.54,68.12 6.63,59.21 6.63,57.95 FRDM1.D14
PWM_BLANK  (via drill 0.61)
  Top 0.254: R1.1 77.04,28.8 79.67,28.8 IC1.23 79.78,28.8 80.7,29.72 81.5,29.72 | 81.5,29.72 88.47,29.72 89.38,28.8 92.7,28.8 IC2.23 | IC4.23 79.67,66.52 79.67,66.06 78.07,64.47 78.07,63.55 77.04,62.52 74.87,62.52 74.18,61.84 74.18,60.92 76.12,58.98 JP12.4 76.01,58.86 74.18,57.04 74.18,54.75 73.61,54.18 v73.61,53.61 | 81.5,29.72 81.5,31.66 80.47,32.69 77.38,32.69 76.35,33.72 76.35,35.43 75.21,36.58 75.21,43.09 v75.32,43.2
  Bottom 0.254: IC4.23 81.15,66.52 84.81,62.75 88.47,62.75 92.13,66.52 92.7,66.52 IC3.23 | v73.61,53.61 73.04,53.61 | 73.04,53.61 70.18,53.61 68.24,55.55 61.04,55.55 60.92,55.44 48.58,55.44 FRDM1.PTC7 | v75.32,43.2 75.09,43.2 73.04,45.26 73.04,53.61
PWM_GSCLK  (via drill 0.61)
  Top 0.254: v90.64,39.32 92.7,41.38 IC2.18 | v68.35,57.49 70.75,57.49 v71.78,58.52 | v72.81,64.81 73.04,65.04 73.04,75.32 77.72,80.01 77.72,81.84 78.75,82.87 80.81,82.87 81.5,82.18 81.5,81.38 79.78,79.67 79.78,79.32 IC4.18
  Bottom 0.254: v90.64,39.32 89.15,37.83 83.78,37.83 80.24,41.38 79.78,41.38 IC1.18 | IC4.18 79.78,79.21 85.27,79.21 86.3,78.18 91.67,78.18 92.7,79.21 IC3.18 | v68.35,57.49 65.15,57.49 64.81,57.84 48.58,57.84 FRDM1.D0 | v71.78,58.52 73.27,58.52 76.12,61.38 JP12.5 | v72.81,64.81 72.81,64.12 75.78,61.15 JP12.5 | IC2.18 92.81,41.49 92.81,41.95 94.41,43.55 94.41,46.86 93.27,48.01 90.53,48.01 88.12,50.41 85.95,50.41 81.61,54.86 81.61,56.69 80.47,57.84 78.75,57.84 78.07,58.52 78.07,59.32 76.12,61.27 JP12.5
PWM_SCLK  (via drill 0.61)
  Top 0.254: 89.72,22.63 91.78,22.63 92.7,23.55 IC2.25 | 89.72,22.63 86.3,22.63 85.38,23.55 79.78,23.55 IC1.25 | IC4.25 79.78,61.38 79.78,61.04 81.5,59.32 81.5,58.52 80.35,57.38 78.64,57.38 78.07,56.81 78.07,55.78 76.12,53.84 JP12.2 | v71.32,56.58 v67.44,56.58 | v89.72,17.95 89.72,22.63 | v51.32,23.09 49.72,23.09 47.55,25.26 47.55,26.98 45.95,28.57 43.43,28.57 42.86,29.15 v42.86,48.23
  Bottom 0.254: IC3.25 92.7,61.38 91.9,61.38 88.35,57.84 83.67,57.84 80.12,61.38 79.78,61.38 IC4.25 | v67.44,56.58 47.89,56.58 47.43,57.04 47.43,58.41 46.86,58.98 37.49,58.98 37.26,58.75 37.26,57.38 36.69,56.81 35.32,56.81 34.75,56.24 34.75,54.52 34.98,54.29 36.69,54.29 37.72,55.32 38.29,55.32 FRDM1.PTC5 38.29,55.21 42.86,50.63 v42.86,48.23 | v71.32,56.58 73.38,54.52 75.44,54.52 76.12,53.84 JP12.2 | v89.72,17.95 89.72,16.23 81.95,8.46 64.24,8.46 55.66,17.03 55.66,18.75 v51.32,23.09
PWM_SIN  (via drill 0.61)
  Top 0.254: v71.44,28.57 71.44,40.58 74.87,44.01 74.87,45.95 v73.95,46.86 73.84,46.86 73.04,46.06 62.41,46.06 62.06,46.41 v61.49,46.41
  Bottom 0.254: v71.44,28.57 71.67,28.57 79.1,21.14 79.67,21.14 IC1.26 | v73.95,46.86 73.95,49.03 76.12,51.21 JP12.1 | v61.49,46.41 53.95,46.41 50.98,49.38 50.98,49.95 49.49,51.44 48.01,51.44 44.92,54.52 44.92,55.78 44.23,56.46 37.49,56.46 36.46,55.44 35.89,55.44 FRDM1.PTC6
PWM_XLAT  (via drill 0.61)
  Top 0.254: IC4.24 79.67,64.01 79.67,63.55 78.07,61.95 78.07,58.29 JP12.3 | IC2.24 92.7,26.06 91.78,25.15 86.3,25.15 85.38,26.06 79.78,26.06 IC1.24 79.67,26.18 77.72,26.18 73.95,29.95 v73.95,39.55 | v56.35,44.58 68.92,44.58 v71.55,41.95
  Bottom 0.254: IC4.24 80.01,64.01 83.55,60.47 88.47,60.47 92.01,64.01 IC3.24 92.7,63.89 94.53,63.89 95.44,62.87 95.44,52.35 96.7,51.09 96.7,46.86 96.24,46.52 96.24,33.49 95.33,32.8 95.33,28.69 92.81,26.18 IC2.24 | v56.35,44.58 55.89,45.03 36.92,45.03 35.32,46.63 35.32,50.41 33.38,52.35 33.38,55.32 FRDM1.PTC10 | v73.95,39.55 v71.55,41.95
TV_SWITCH
  Top 0.254: R39.2 1.83,71.67 3.2,71.67 13.03,61.84 13.03,60.69 14.74,58.98 15.66,58.98 16.69,57.95 FRDM1.D12
(copper drawn outside any net)
  shapes: Top area x1

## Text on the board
tNames: SMALL LED/OPTO | NC | 5B | 5G | 5R | 2B | 2G | 2R | 1B | 1G | 1R | Prt48 | Prt47 | Prt46 | Prt21 | +5V | GND | GND | +12V | Prt45 | LAMPS/STROBE | +5V | LED6 | 4G | 4G | 4R | 3B | 3G | 3R | 2ND PSU | Prt20 | Prt19 | Prt18 | Prt17 | 3G | +5V | 3R | 5B | 2B | 5G | 2G | 5R | Prt44 | Prt43 | 2R | 4B | RGB FLASHERS | Prt42 | Prt41 | 1B | 4G | Prt40 | Prt39 | 1G | HI POWER OUTS | +5V | 4R | PC PSU | SOUT | Prt38 | Prt37 | +5V | 1R | 3B | GSCLK | Prt36 | Prt35 | BLANK | Prt34 | Prt33 | XLAT | SCLK | SIN | Prt32 | Prt31 | Prt30 | Prt29 | Prt28 | Prt27 | HI POWER OUTS | Prt26 | Prt25 | Prt24 | Prt23 | Prt22 | TV ON | TV2 | TV1 | Prt21 / KNOCKER | PINSCAPE Expansion Board / B1 Nov2015 | TIMER BYPASS | NC | 23 | 21 | 19 | 17 | 15 | 13 | 11 | 9 | 7 | 5 | 3 | 1 | +Led | -Led | +5V | Vcc | PTE21 | PTB0 | Common | 24 | 22 | 20 | BUTTON INPUTS | 8 | 6 | 4 | 2 | CAL BTN | PLUNGER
